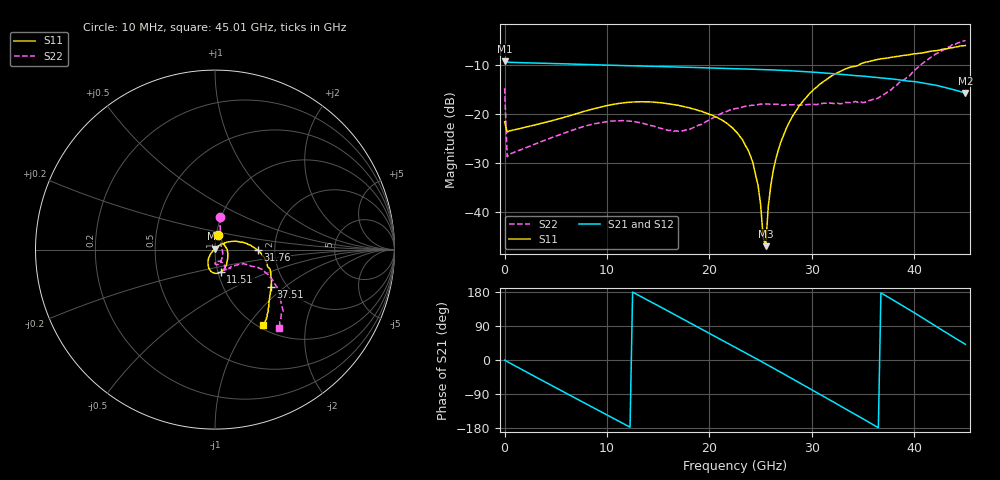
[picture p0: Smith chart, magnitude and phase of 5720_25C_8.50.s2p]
! Device:  ADRF5720
! Description: 0.5dB LSB GaAs MMIC 6-bit Digital Attenuator
! Frequency:  0.000009 -  40 GHz
! Ports:
!	RF1	= Port 1
!	RF2	= Port 2
! Vdd:  3.3 Volt
! Vss:  -3.3 Volt
! Control:  0/3.3 Volt
! State:  8.50 dB attenuation
! Data:  The device was measured using G-S-G Probes on a matrix board.
!  Data was collected using an calibrated 4 port network analyzer.
!  The reference plane for this measurement is at the launchers.
! Note:  Analog Devices supplies this data as a sample of measured data
!  for this product.  Your particular data for this product may vary.
!  Data was taken at 25 degrees C.
!  Analog Devices reserves the right to change this data at anytime.
# GHZ S DB R 45.0
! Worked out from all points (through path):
!   181 points, 10 MHz to 45.01 GHz, reference 45 ohm
!   highest |S21| = -9.25 dB at 10 MHz (marker M1); lowest = -15.7 dB at 45.01 GHz (marker M2)
!   group delay of S21, straight-line fit = 41.5 ps
!   lowest |S11| = -47.1 dB at 25.51 GHz (marker M3), VSWR 1.01, Z = 45 + j0.397 ohm
!   |S11| at or under -10 dB: start of sweep to 34.61 GHz
!   |S22| runs from -28.8 to -5.0 dB; largest |S21 - S12| = 0.00043
!   S11 on the Smith chart (normalised r, x): 10 MHz: 1.02, +0.17; 11.51 GHz: 1.03, -0.26; 31.76 GHz: 1.62, -0.01; 37.51 GHz: 1.66, -0.80; 45.01 GHz: 1.05, -1.18
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0.01  -21.64 79.0  -9.25 -0.5  -9.26 -0.5  -14.74 82.0
0.26  -23.72 5.3  -9.43 -4.0  -9.44 -4.0  -28.76 10.2
4.26  -21.60 -31.2  -9.67 -62.4  -9.68 -62.4  -25.14 -41.9
7.76  -19.50 -53.2  -9.88 -112.7  -9.88 -112.7  -22.57 -65.1
11.51  -17.77 -75.3  -10.12 -166.5  -10.12 -166.5  -21.38 -83.5
15.26  -17.72 -94.5  -10.32 139.5  -10.32 139.5  -22.95 -87.8
19.01  -19.37 -108.8  -10.54 85.2  -10.54 85.2  -22.27 -62.7
22.76  -23.97 -125.5  -10.78 30.4  -10.78 30.4  -18.87 -61.2
24.26  -30.01 -137.5  -10.88 8.3  -10.88 8.3  -18.25 -64.4
24.76  -34.62 -142.5  -10.90 0.9  -10.91 0.9  -18.10 -65.4
25.26  -45.26 -177.0  -10.94 -6.6  -10.94 -6.6  -18.03 -66.7
25.51  -47.08 84.7  -10.96 -10.3  -10.96 -10.3  -17.96 -67.1
25.76  -38.88 62.4  -10.98 -14.1  -10.98 -14.0  -17.99 -67.0
26.01  -34.60 50.0  -11.00 -17.8  -11.00 -17.8  -18.07 -67.4
26.76  -27.25 41.3  -11.06 -29.1  -11.06 -29.1  -18.04 -66.8
28.26  -20.04 27.0  -11.22 -51.8  -11.22 -51.8  -18.14 -66.9
30.26  -14.90 10.9  -11.48 -82.4  -11.48 -82.3  -18.06 -62.6
31.76  -12.50 -0.5  -11.72 -105.2  -11.72 -105.2  -17.79 -59.2
37.51  -8.54 -33.7  -12.79 165.3  -12.80 165.3  -15.36 -28.1
37.76  -8.42 -34.8  -12.84 161.4  -12.84 161.4  -15.07 -26.5
41.26  -7.35 -45.6  -13.80 103.9  -13.81 104.0  -9.03 -27.0
45.01  -6.01 -57.6  -15.74 41.4  -15.74 41.5  -4.98 -50.5
